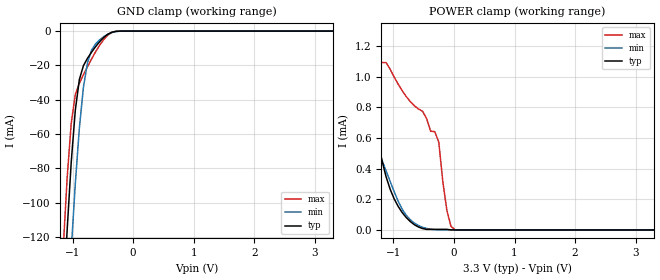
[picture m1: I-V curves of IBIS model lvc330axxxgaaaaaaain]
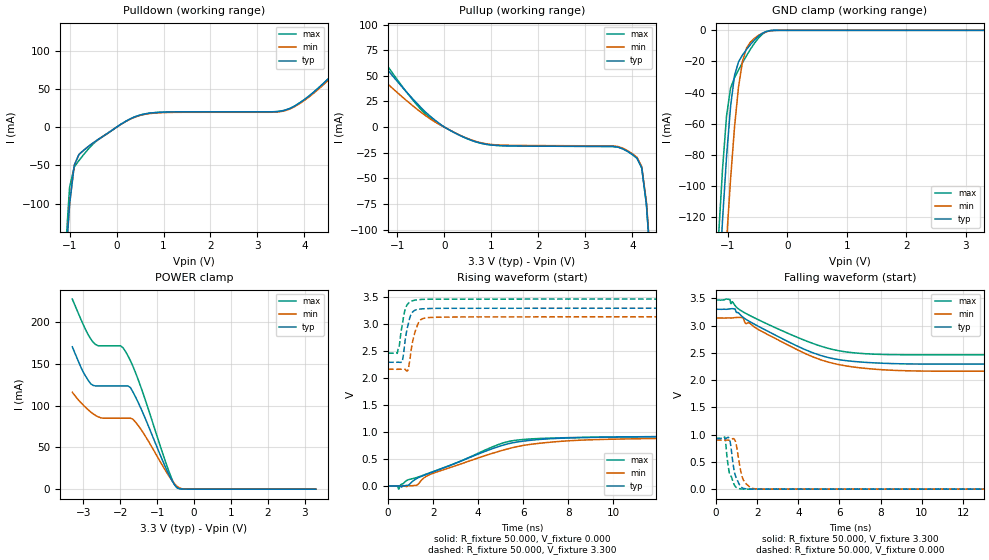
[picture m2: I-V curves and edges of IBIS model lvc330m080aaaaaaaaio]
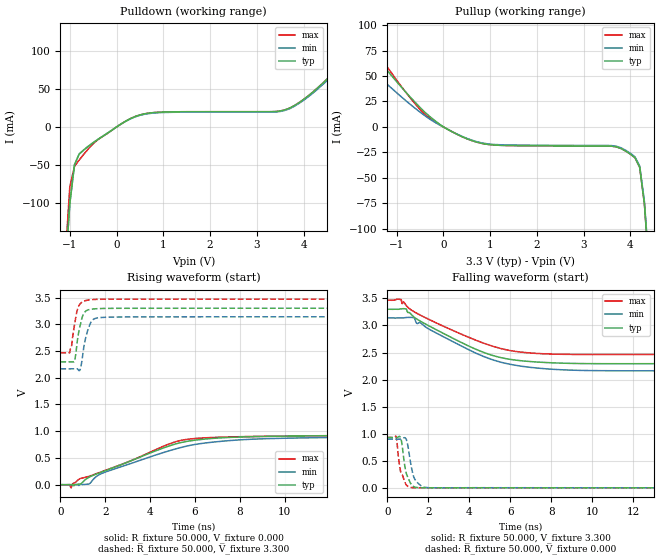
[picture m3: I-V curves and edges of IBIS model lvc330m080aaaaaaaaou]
| IBIS Models Generator: Lattice Radiant Software (64-bit) 2023.1.1.200.1
| Report Generate Date: Nov 30 2023
| Report Generate Time: 09:30:31
| IBIS File LibisMaker.ibs
| Cadence Design Systems, Inc. 2022
[IBIS ver]   4.2
[File Name]   LAB04_Async_rst.ibs
[File Rev]   1.7
[Date]   Wed Dec 14 00:26:56 PST 2022
[Source]   Lattice Semiconductor 28fdsoi Process
[Notes]   Device: LFCPNX-100 Final
   Lattice Semiconductor has worked hard to ensure the
   models below are accurate and complete.  However, the
   data below was generated using simulation of the
   input/output model files for the silicon.  Therefore,
   the data below is for reference and initial design
   purposes only.
   Lattice Semiconductor grants permission to use this
   data for use in printed circuit design using this
   Lattice programmable logic device.  Other use of this
   code, including the selling or duplication of any
   portion is strictly prohibited.
|   NAMING CONVENTION
   The IBIS [Model] header is limited by the specification to a
   total of characters.  With such a set of characters available
   for naming models it becomes important to attempt to
   meaningfully encode the IO standards so they fit within the
   twenty character limit.  It would seem that twenty characters
   would provide room enough for describing IO's.  However, the
   PLD IO structure continues to grow more and more complex.  The
   complexity is making the twenty characters insuffiently
   descriptive.  In order to overcome this issue the naming
   convention described below is implemented to resolve the issue.
The twenty character space is managed as follows:
   bbbvvvsdddprttmaoixx
   b = standard
   v = voltage (x.xx V)
   s = slew code
   d = drive (xx.x ma)
   p = pullmode code
   r = impedance
   t = termination code
   m = mipi hard dphy mode
   o = diff resistor code
   i = diff  current code
   x = reserved
   standard
   LVCMOS   lvc
   LVCMOSH   lvh
   LVCMOSR   lvr
   LVCMOSD   lvd
   LVTTL   lvt
   lvttld   ltd
   sstl_I   ss1
   sstl_II   ss2
   sstld_I   s1d
   sstld_II   s2d
   hsul   hs1
   hsuld   h1d
   hstl_I   hs1
   hstld_I   h1d
   lvds   lvs
   lvdse   lve
   SUBLVDS   slv
   sublvdse   sle
   sublvdseh   slh
   slvs   svs
   mipi   mip
   vref1   vr1
   lvstl_I   ll1
   lvstl_II   ll2
   lvstld_I   l1d
   lvstld_II   l2d
   slew
   na   a
   fast   f
   slow   s
   med   m
   drive
   2   020
   4   040
   6   060
   8   080
   10   100
   12   120
   16   160
   50rs   r50
   na   xxx
   pullmode/clamp on
   none   a/e
   failsafe   a/e
   up   b/f
   down   c/g
   keeper   d/h
   i3c   i
   impedance
   off   a
   termination
   off   aa
   40   bb
   50   cc
   60   dd
   75   ee
   150   ff
   48   gg
   80   hh
   120   ii
   mipi hard dphy mode
   off   a
   lp   l
   hs   h
   differential resistor
   off   a
   100   b
   differential current
   NA   a
   2.0   b
   3.5   c
   Reserved   IO type
   in   input only (mipi: rx)
   ou   output (mipi: tx)
   io   I/O
   od   Open drain
   on   Inverting differential I/O
  (signal name only)
   op   Non-Inverting differential I/O
  (signal name only)
  (signal name only)
   All the IO models are generated with pull mode set to none.
   Lattice Semiconductor Corporation
   5555 NE Moore Court
   Hillsboro, OR 97214
   U.S.A
   TEL: 1-800-Lattice (USA and Canada)
   408-826-6000 (other locations)
   web: http://www.latticesemi.com/
   email: techsupport@latticesemi.com
[Disclaimer] This IBIS source code is intended as a design reference
   which illustrates how the Lattice Semiconductor device operates.
   It is the user's responsibility to verify their design for
   consistency and functionality through the use of formal
   verification methods.  Lattice Semiconductor provides no warranty
   regarding the use or functionality of this data.
[Copyright]   Copyright 2022 by Lattice Semiconductor Corporation
|   Component LFCPNX
[Component] LFCPNX
[Manufacturer] Lattice Semiconductor Corp.
[Package]
|LFG672
| variable   typ   min   max
R_pkg   0.85482   0.28979   1.626
L_pkg   4.948e-9   1.752e-9   8.572e-9
C_pkg   1.721e-12   9.177e-13   2.607e-12
[Pin]  signal_name   model_name   R_pin   L_pin   C_pin
L9   TDI   lvc330axxxgaaaaaaain
M5   TCK   lvc330axxxgaaaaaaain
L7   TMS   lvc330axxxgaaaaaaain
M8   TDO   lvc330m080aaaaaaaaio
R9   LED4   lvc330m080aaaaaaaaou
R8   LED3   lvc330m080aaaaaaaaou
R4   LED2   lvc330m080aaaaaaaaou
R5   LED1   lvc330m080aaaaaaaaou
W21   en   lvh180axxxgaaaaaaain
N9   reset   lvc330axxxgaaaaaaain
| Models and submodels in the file (4): lvc330axxxgaaaaaaain (Input), lvc330m080aaaaaaaaio (I/O), lvc330m080aaaaaaaaou (Output), lvh180axxxgaaaaaaain (Input)
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[Model] lvc330axxxgaaaaaaain
Model_type Input
Polarity   Non-Inverting
Enable   Active-High
Vinl =  0.800V
Vinh =  2.000V
C_comp   5.000pF   4.000pF   5.500pF
[Temperature Range]   25.000   0.125k   -40.000
[Voltage Range]   3.300V   3.140V   3.470V
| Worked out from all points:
|   GND clamp passes 1 mA (typ) near -0.37 V on its own axis
|   POWER clamp passes 1 mA (typ) near -1.47 V on its own axis
[GND_clamp]
|Voltage   I(typ)   I(min)   I(max)
-3.3V     -1.865A    -1.847A    -1.883A
-1.156V   -160.1mA   -214.1mA   -127.6mA
-1.089V   -115.7mA   -169.6mA   -85.35mA
-1.022V   -76.45mA   -127.5mA   -53.7mA
-955mV    -46.24mA   -89.13mA   -37.05mA
-888mV    -28.3mA    -56.66mA   -30.41mA
-821mV    -20.19mA   -32.82mA   -25.49mA
-754mV    -15.89mA   -18.49mA   -20.81mA
-620mV    -9.094mA   -7.515mA   -12.09mA
-419mV    -1.868mA   -1.846mA   -2.383mA
-218mV    -16.48uA   -78.61uA   -6.639uA
3.3V      0A         0A         0A
[POWER_clamp]
|Voltage   I(typ)   I(min)   I(max)
-3.3V     37.53mA    9.364mA    73.7mA
-1.792V   1.823mA    1.318mA    2.466mA
-1.591V   1.29mA     991.8uA    1.714mA
-1.457V   981.8uA    795.4uA    1.299mA
-1.39V    843.7uA    703.6uA    1.091mA
-1.122V   347.7uA    385.2uA    1.091mA
-854mV    112.9uA    134.5uA    907uA
-586mV    19.15uA    28.85uA    788.2uA
-251mV    3.861uA    1.254uA    573.3uA
-117mV    3.861uA    1.254uA    126.7uA
17mV      69.96nA    1.254uA    1.636uA
3.3V      0A         0A         0A
[Model] lvc330m080aaaaaaaaio
Model_type I/O
Polarity   Non-Inverting
Enable   Active-Low
Vinl =  0.800V
Vinh =  2.000V
Vmeas =  1.650V
Cref =  0.0F
Rref =  1.000M
Vref =  0.0V
C_comp   5.000pF   4.000pF   5.500pF
[Temperature Range]   25.000   0.125k   -40.000
[Voltage Range]   3.300V   3.140V   3.470V
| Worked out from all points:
|   slope of the pulldown table from 0 to 0.495 V, typ, clamps not added: 31.5 ohm
|   slope of the pullup table from 0 to 0.495 V, typ, clamps not added: 43.2 ohm
|   GND clamp passes 1 mA (typ) near -0.37 V on its own axis
|   POWER clamp passes 1 mA (typ) near -0.42 V on its own axis
|   rising waveform, R_fixture 50.000, V_fixture 0.000: 20-80 % time 3.47ns typ, 3.91ns min, 3.27ns max; typ from 0 V to 0.929 V
|   rising waveform, R_fixture 50.000, V_fixture 3.300: 20-80 % time 248ps typ, 295ps min, 236ps max; typ from 2.3 V to 3.3 V
|   falling waveform, R_fixture 50.000, V_fixture 3.300: 20-80 % time 3.22ns typ, 3.2ns min, 3.51ns max; typ from 3.3 V to 2.3 V
|   falling waveform, R_fixture 50.000, V_fixture 0.000: 20-80 % time 273ps typ, 284ps min, 288ps max; typ from 0.929 V to 0 V
[GND_clamp]
|Voltage   I(typ)   I(min)   I(max)
-3.3V     -1.887A    -1.873A    -1.902A
-1.156V   -166.9mA   -224mA     -132.1mA
-1.089V   -121.5mA   -178.4mA   -88.64mA
-1.022V   -81.05mA   -135.2mA   -54.94mA
-955mV    -48.98mA   -95.79mA   -37.15mA
-888mV    -28.98mA   -62.05mA   -30.42mA
-821mV    -20.23mA   -36.35mA   -25.49mA
-754mV    -15.89mA   -19.89mA   -20.81mA
-687mV    -12.34mA   -11.44mA   -16.31mA
-620mV    -9.094mA   -7.515mA   -12.09mA
-419mV    -1.869mA   -1.836mA   -2.383mA
3.3V      0A         0A         0A
[POWER_clamp]
|Voltage   I(typ)   I(min)   I(max)
-3.3V     170.3mA    115.9mA    227.4mA
-2.998V   139.6mA    100.3mA    196.3mA
-2.797V   125.9mA    92.2mA     179.4mA
-2.596V   123.5mA    86.45mA    171.5mA
-1.993V   123.5mA    84.93mA    171.5mA
-1.792V   123.5mA    84.93mA    159.6mA
-1.658V   116.4mA    83.68mA    147.1mA
-1.457V   98.28mA    72.65mA    124.1mA
-720mV    21.08mA    18.41mA    25.96mA
-452mV    1.573mA    3.148mA    1.229mA
-184mV    5.589uA    37.85uA    1.612uA
3.3V      0A         0A         0A
[Pulldown]
|Voltage   I(typ)   I(min)   I(max)
-3.3V     -3.025A    -3.025A    -3.918A
-1.1V     -192.9mA   -192.9mA   -175.3mA
-1V       -101.2mA   -101.2mA   -78.95mA
-900mV    -49.86mA   -49.86mA   -52.21mA
-800mV    -35.81mA   -35.81mA   -43.74mA
200mV     7.775mA    7.542mA    7.775mA
800mV     18.91mA    18.34mA    18.91mA
3.6V      22.45mA    21.77mA    22.45mA
4.1V      40.8mA     39.58mA    40.8mA
5.4V      113.7mA    110.3mA    113.7mA
6.1V      131.6mA    127.7mA    131.6mA
6.6V      184.5mA    179mA      184.5mA
[Pullup]
|Voltage   I(typ)   I(min)   I(max)
-3.3V     145.5mA    90.7mA     185.8mA
-2.7V     96.8mA     74.7mA     125.4mA
-2.1V     95.1mA     70.11mA    105.4mA
-1.8V     86.3mA     64.15mA    96.9mA
-500mV    19.13mA    14.57mA    17.21mA
0V        28.62nA    228.6nA    28.62nA
600mV     -13.29mA   -12.89mA   -13.29mA
3.9V      -23.67mA   -22.96mA   -23.67mA
4.2V      -39.73mA   -38.54mA   -39.73mA
4.3V      -75.4mA    -73.1mA    -75.4mA
4.4V      -140.5mA   -136.3mA   -140.5mA
6.6V      -2.178A    -2.113A    -2.178A
[Ramp]
| variable   typ   min   max
dV/dt_r   0.789/3.474n   0.590/3.936n   0.521/3.276n
dV/dt_f   0.706/3.253n   0.547/3.212n   0.513/3.516n
R_load = 50.000
[Rising Waveform]
R_fixture = 50.000
V_fixture = 0.000
V_fixture_min = 0.000
V_fixture_max = 0.000
|  time   V(typ)   V(min)   V(max)
0s        488.9uV    1.198mV    488.9uV
395ps     637.6uV    952.2uV    3.238mV
475ps     718.1uV    1.204mV    -58.62mV
816ps     11.39mV    -13.02mV   99.9mV
1.256ns   135.1mV    11.8mV     155.5mV
2.016ns   265mV      239.2mV    270.5mV
4.885ns   729.4mV    638.7mV    767.7mV
5.78ns    819.5mV    735.4mV    854.8mV
9.109ns   902.9mV    859.8mV    905.4mV
20ns      929.1mV    899.7mV    931mV
[Rising Waveform]
R_fixture = 50.000
V_fixture = 3.300
V_fixture_min = 3.140
V_fixture_max = 3.470
|  time   V(typ)   V(min)   V(max)
0s        2.297V     2.167V     2.467V
409ps     2.297V     2.166V     2.466V
616ps     2.299V     2.168V     2.961V
734ps     2.622V     2.168V     3.237V
866ps     2.953V     2.141V     3.375V
1.036ns   3.197V     2.555V     3.43V
1.276ns   3.274V     2.953V     3.455V
1.486ns   3.287V     3.096V     3.463V
2.077ns   3.297V     3.131V     3.469V
20ns      3.3V       3.14V      3.47V
[Falling Waveform]
R_fixture = 50.000
V_fixture = 3.300
V_fixture_min = 3.140
V_fixture_max = 3.470
|  time   V(typ)   V(min)   V(max)
0s        3.3V       3.14V      3.47V
666ps     3.307V     3.141V     3.481V
726ps     3.309V     3.14V      3.403V
924ps     3.306V     3.147V     3.369V
1.275ns   3.165V     3.146V     3.261V
1.436ns   3.12V      3.04V      3.227V
4.236ns   2.575V     2.505V     2.741V
6.39ns    2.354V     2.256V     2.514V
9.897ns   2.295V     2.167V     2.465V
20ns      2.297V     2.167V     2.467V
[Falling Waveform]
R_fixture = 50.000
V_fixture = 0.000
V_fixture_min = 0.000
V_fixture_max = 0.000
|  time   V(typ)   V(min)   V(max)
0s        929.1mV    899.7mV    931mV
432ps     928.7mV    899.2mV    951mV
635ps     935.9mV    899.2mV    328.3mV
704ps     834.8mV    904.4mV    247.5mV
846ps     423.4mV    926.9mV    115mV
936ps     256.3mV    884.1mV    51.1mV
1.193ns   51.59mV    350.2mV    4.707mV
1.432ns   6.847mV    110.5mV    217.4uV
1.966ns   398.9uV    3.886mV    -527.1uV
20ns      488.9uV    1.198mV    488.9uV
[Model] lvc330m080aaaaaaaaou
Model_type Output
Polarity   Non-Inverting
Enable   Active-High
Vmeas =  1.650V
Cref =  0.0F
Rref =  1.000M
Vref =  0.0V
C_comp   5.000pF   4.000pF   5.500pF
[Temperature Range]   25.000   0.125k   -40.000
[Voltage Range]   3.300V   3.140V   3.470V
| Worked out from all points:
|   slope of the pulldown table from 0 to 0.495 V, typ, clamps not added: 31.5 ohm
|   slope of the pullup table from 0 to 0.495 V, typ, clamps not added: 43.2 ohm
|   rising waveform, R_fixture 50.000, V_fixture 0.000: 20-80 % time 3.47ns typ, 3.91ns min, 3.27ns max; typ from 0 V to 0.929 V
|   rising waveform, R_fixture 50.000, V_fixture 3.300: 20-80 % time 248ps typ, 295ps min, 236ps max; typ from 2.3 V to 3.3 V
|   falling waveform, R_fixture 50.000, V_fixture 3.300: 20-80 % time 3.22ns typ, 3.2ns min, 3.51ns max; typ from 3.3 V to 2.3 V
|   falling waveform, R_fixture 50.000, V_fixture 0.000: 20-80 % time 273ps typ, 284ps min, 288ps max; typ from 0.929 V to 0 V
[Pulldown]
|Voltage   I(typ)   I(min)   I(max)
-3.3V     -3.025A    -3.025A    -3.918A
-1.1V     -192.9mA   -192.9mA   -175.3mA
-1V       -101.2mA   -101.2mA   -78.95mA
-900mV    -49.86mA   -49.86mA   -52.21mA
-800mV    -35.81mA   -35.81mA   -43.74mA
200mV     7.775mA    7.542mA    7.775mA
800mV     18.91mA    18.34mA    18.91mA
3.6V      22.45mA    21.77mA    22.45mA
4.1V      40.8mA     39.58mA    40.8mA
5.4V      113.7mA    110.3mA    113.7mA
6.1V      131.6mA    127.7mA    131.6mA
6.6V      184.5mA    179mA      184.5mA
[Pullup]
|Voltage   I(typ)   I(min)   I(max)
-3.3V     145.5mA    90.7mA     185.8mA
-2.7V     96.8mA     74.7mA     125.4mA
-2.1V     95.1mA     70.11mA    105.4mA
-1.8V     86.3mA     64.15mA    96.9mA
-500mV    19.13mA    14.57mA    17.21mA
0V        28.62nA    228.6nA    28.62nA
600mV     -13.29mA   -12.89mA   -13.29mA
3.9V      -23.67mA   -22.96mA   -23.67mA
4.2V      -39.73mA   -38.54mA   -39.73mA
4.3V      -75.4mA    -73.1mA    -75.4mA
4.4V      -140.5mA   -136.3mA   -140.5mA
6.6V      -2.178A    -2.113A    -2.178A
[Ramp]
| variable   typ   min   max
dV/dt_r   0.789/3.474n   0.590/3.936n   0.521/3.276n
dV/dt_f   0.706/3.253n   0.547/3.212n   0.513/3.516n
R_load = 50.000
[Rising Waveform]
R_fixture = 50.000
V_fixture = 0.000
V_fixture_min = 0.000
V_fixture_max = 0.000
|  time   V(typ)   V(min)   V(max)
0s        488.9uV    1.198mV    488.9uV
395ps     637.6uV    952.2uV    3.238mV
475ps     718.1uV    1.204mV    -58.62mV
816ps     11.39mV    -13.02mV   99.9mV
1.256ns   135.1mV    11.8mV     155.5mV
2.016ns   265mV      239.2mV    270.5mV
4.885ns   729.4mV    638.7mV    767.7mV
5.78ns    819.5mV    735.4mV    854.8mV
9.109ns   902.9mV    859.8mV    905.4mV
20ns      929.1mV    899.7mV    931mV
[Rising Waveform]
R_fixture = 50.000
V_fixture = 3.300
V_fixture_min = 3.140
V_fixture_max = 3.470
|  time   V(typ)   V(min)   V(max)
0s        2.297V     2.167V     2.467V
409ps     2.297V     2.166V     2.466V
616ps     2.299V     2.168V     2.961V
734ps     2.622V     2.168V     3.237V
866ps     2.953V     2.141V     3.375V
1.036ns   3.197V     2.555V     3.43V
1.276ns   3.274V     2.953V     3.455V
1.486ns   3.287V     3.096V     3.463V
2.077ns   3.297V     3.131V     3.469V
20ns      3.3V       3.14V      3.47V
[Falling Waveform]
R_fixture = 50.000
V_fixture = 3.300
V_fixture_min = 3.140
V_fixture_max = 3.470
|  time   V(typ)   V(min)   V(max)
0s        3.3V       3.14V      3.47V
666ps     3.307V     3.141V     3.481V
726ps     3.309V     3.14V      3.403V
924ps     3.306V     3.147V     3.369V
1.275ns   3.165V     3.146V     3.261V
1.436ns   3.12V      3.04V      3.227V
4.236ns   2.575V     2.505V     2.741V
6.39ns    2.354V     2.256V     2.514V
9.897ns   2.295V     2.167V     2.465V
20ns      2.297V     2.167V     2.467V
[Falling Waveform]
R_fixture = 50.000
V_fixture = 0.000
V_fixture_min = 0.000
V_fixture_max = 0.000
|  time   V(typ)   V(min)   V(max)
0s        929.1mV    899.7mV    931mV
432ps     928.7mV    899.2mV    951mV
635ps     935.9mV    899.2mV    328.3mV
704ps     834.8mV    904.4mV    247.5mV
846ps     423.4mV    926.9mV    115mV
936ps     256.3mV    884.1mV    51.1mV
1.193ns   51.59mV    350.2mV    4.707mV
1.432ns   6.847mV    110.5mV    217.4uV
1.966ns   398.9uV    3.886mV    -527.1uV
20ns      488.9uV    1.198mV    488.9uV
